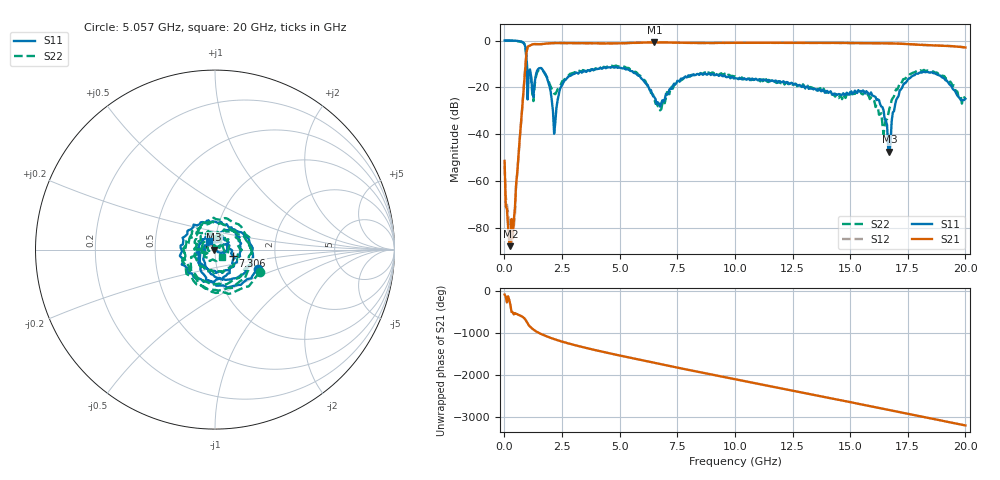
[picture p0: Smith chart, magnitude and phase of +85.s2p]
!Agilent Technologies,E8361C,US49010292,A.09.42.06
!Agilent E8361C: A.09.42.06
!Date: Wednesday, July 09, 2025 01:42:58
!Correction: S11(Full 2 Port(1,2))
!S21(Full 2 Port(1,2))
!S12(Full 2 Port(1,2))
!S22(Full 2 Port(1,2))
!S2P File: Measurements: S11, S21, S12, S22:
# Hz S  dB  R 50
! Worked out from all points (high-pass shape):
!   401 points, 10 MHz to 20 GHz, reference 50 ohm
!   highest |S21| = -0.77 dB at 6.507 GHz (marker M1); lowest = -87.7 dB at 259.9 MHz (marker M2)
!   |S21| within 3 dB of the highest: 988 MHz to end of sweep
!   lowest |S11| = -47.4 dB at 16.7 GHz (marker M3), VSWR 1.01, Z = 49.6 + j0.0435 ohm
!   |S11| at or under -10 dB: 965 MHz to end of sweep
!   |S22| runs from -40.0 to 0.0 dB; largest |S21 - S12| = 0.011
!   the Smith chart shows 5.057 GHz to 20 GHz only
!   S11 on the Smith chart (normalised r, x): 5.057 GHz: 1.57, -0.37; 7.306 GHz: 1.22, -0.09; 20 GHz: 0.93, +0.09
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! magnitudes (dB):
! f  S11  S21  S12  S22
! 10 MHz  0.0  -51.4  -53.7  -0.1
! 259.9 MHz  0.0  -87.7  -76.9  0.0
! 409.8 MHz  -0.1  -76.7  -79.5  -0.1
! 809.6 MHz  -0.8  -24.1  -24.1  -0.9
! 1.059 GHz  -12.7  -2.3  -2.4  -13.1
! 1.259 GHz  -24.1  -1.5  -1.6  -25.8
! 1.709 GHz  -13.2  -1.4  -1.4  -13.3
! 2.209 GHz  -34.9  -1.1  -1.1  -22.9
! 2.559 GHz  -17.9  -1.1  -1.1  -17.2
! 3.358 GHz  -13.7  -1.1  -1.1  -13.2
! 5.057 GHz  -11.6  -1.2  -1.2  -11.0
! 6.507 GHz  -24.1  -0.8  -0.8  -24.9
! 6.707 GHz  -26.9  -0.8  -0.8  -28.1
! 7.306 GHz  -19.5  -0.9  -0.9  -20.5
! 10.01 GHz  -16.0  -1.0  -1.0  -15.3
! 13.35 GHz  -20.5  -1.0  -1.0  -20.1
! 16 GHz  -23.5  -1.1  -1.1  -25.8
! 16.5 GHz  -33.7  -1.2  -1.2  -35.9
! 16.7 GHz  -47.4  -1.2  -1.2  -29.1
! 17.1 GHz  -23.7  -1.3  -1.3  -19.6
! 17.8 GHz  -14.8  -1.7  -1.7  -13.6
! 20 GHz  -24.9  -3.0  -2.9  -24.9
